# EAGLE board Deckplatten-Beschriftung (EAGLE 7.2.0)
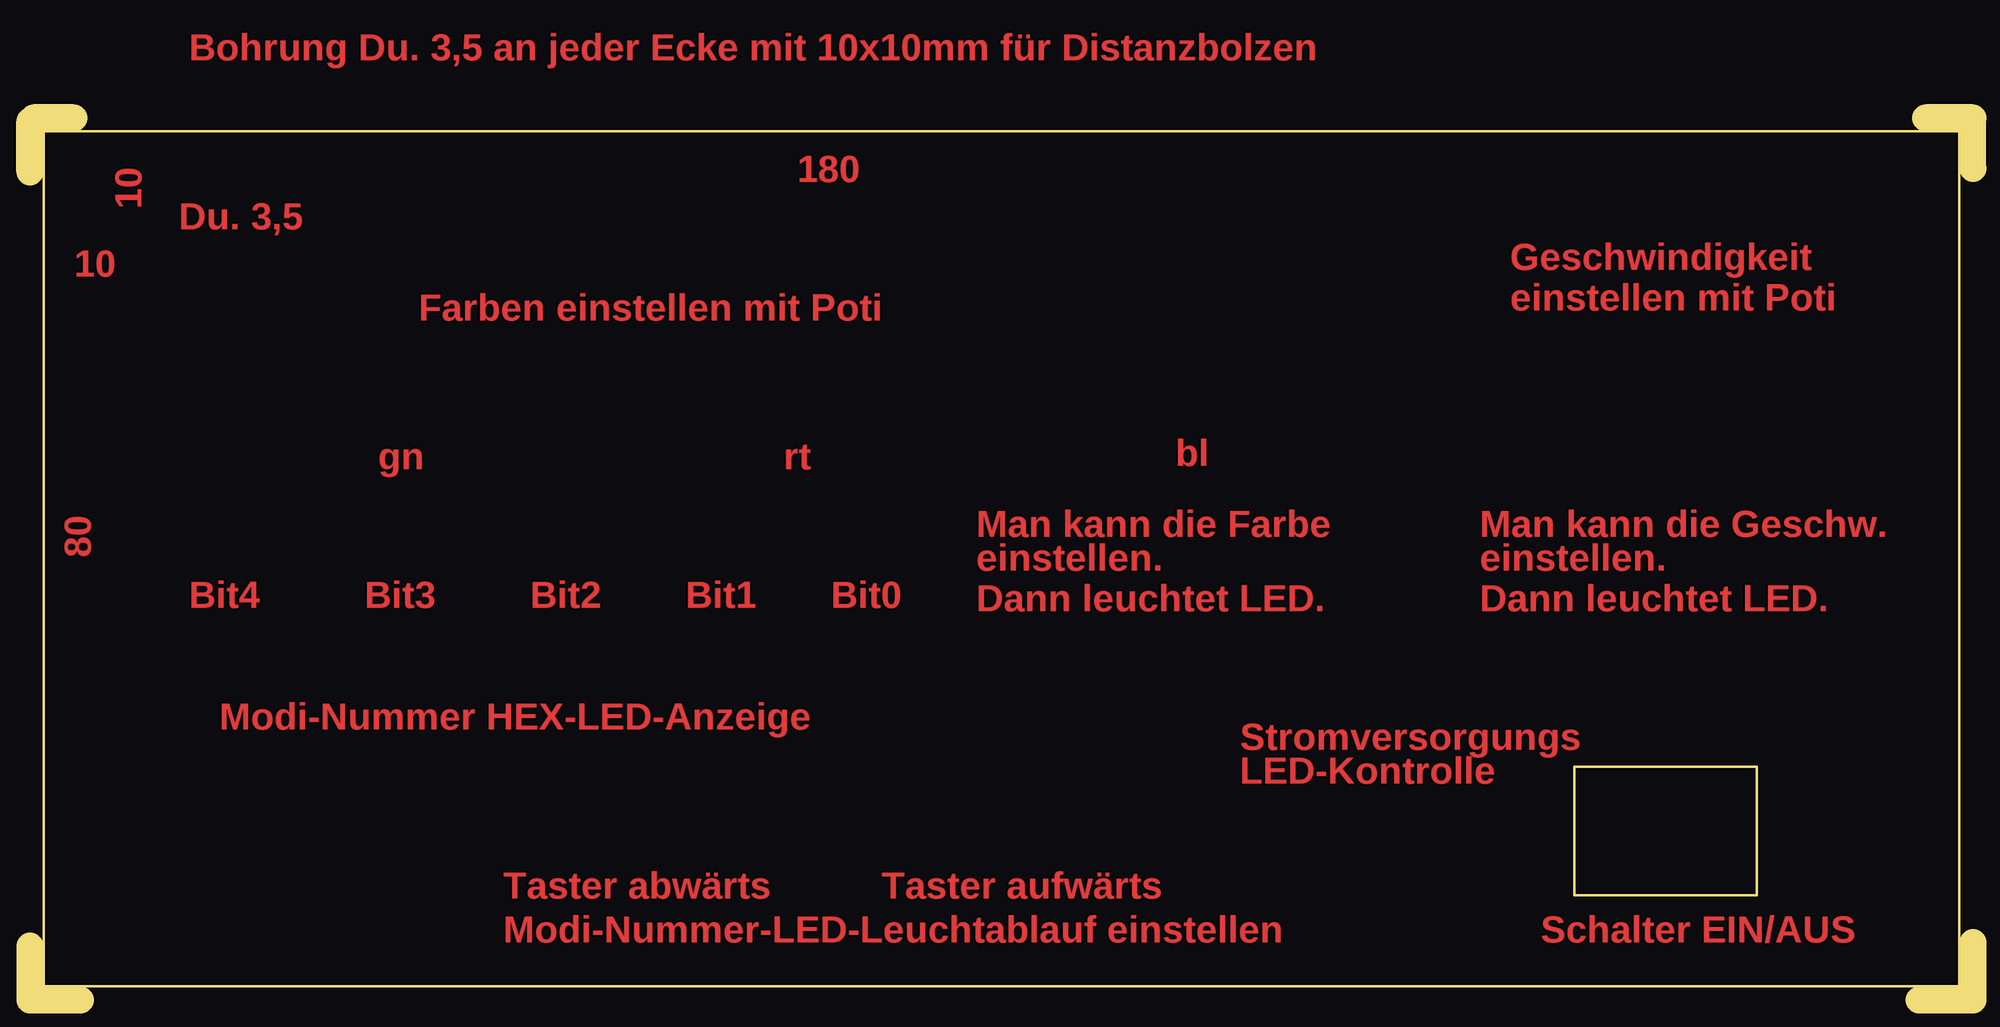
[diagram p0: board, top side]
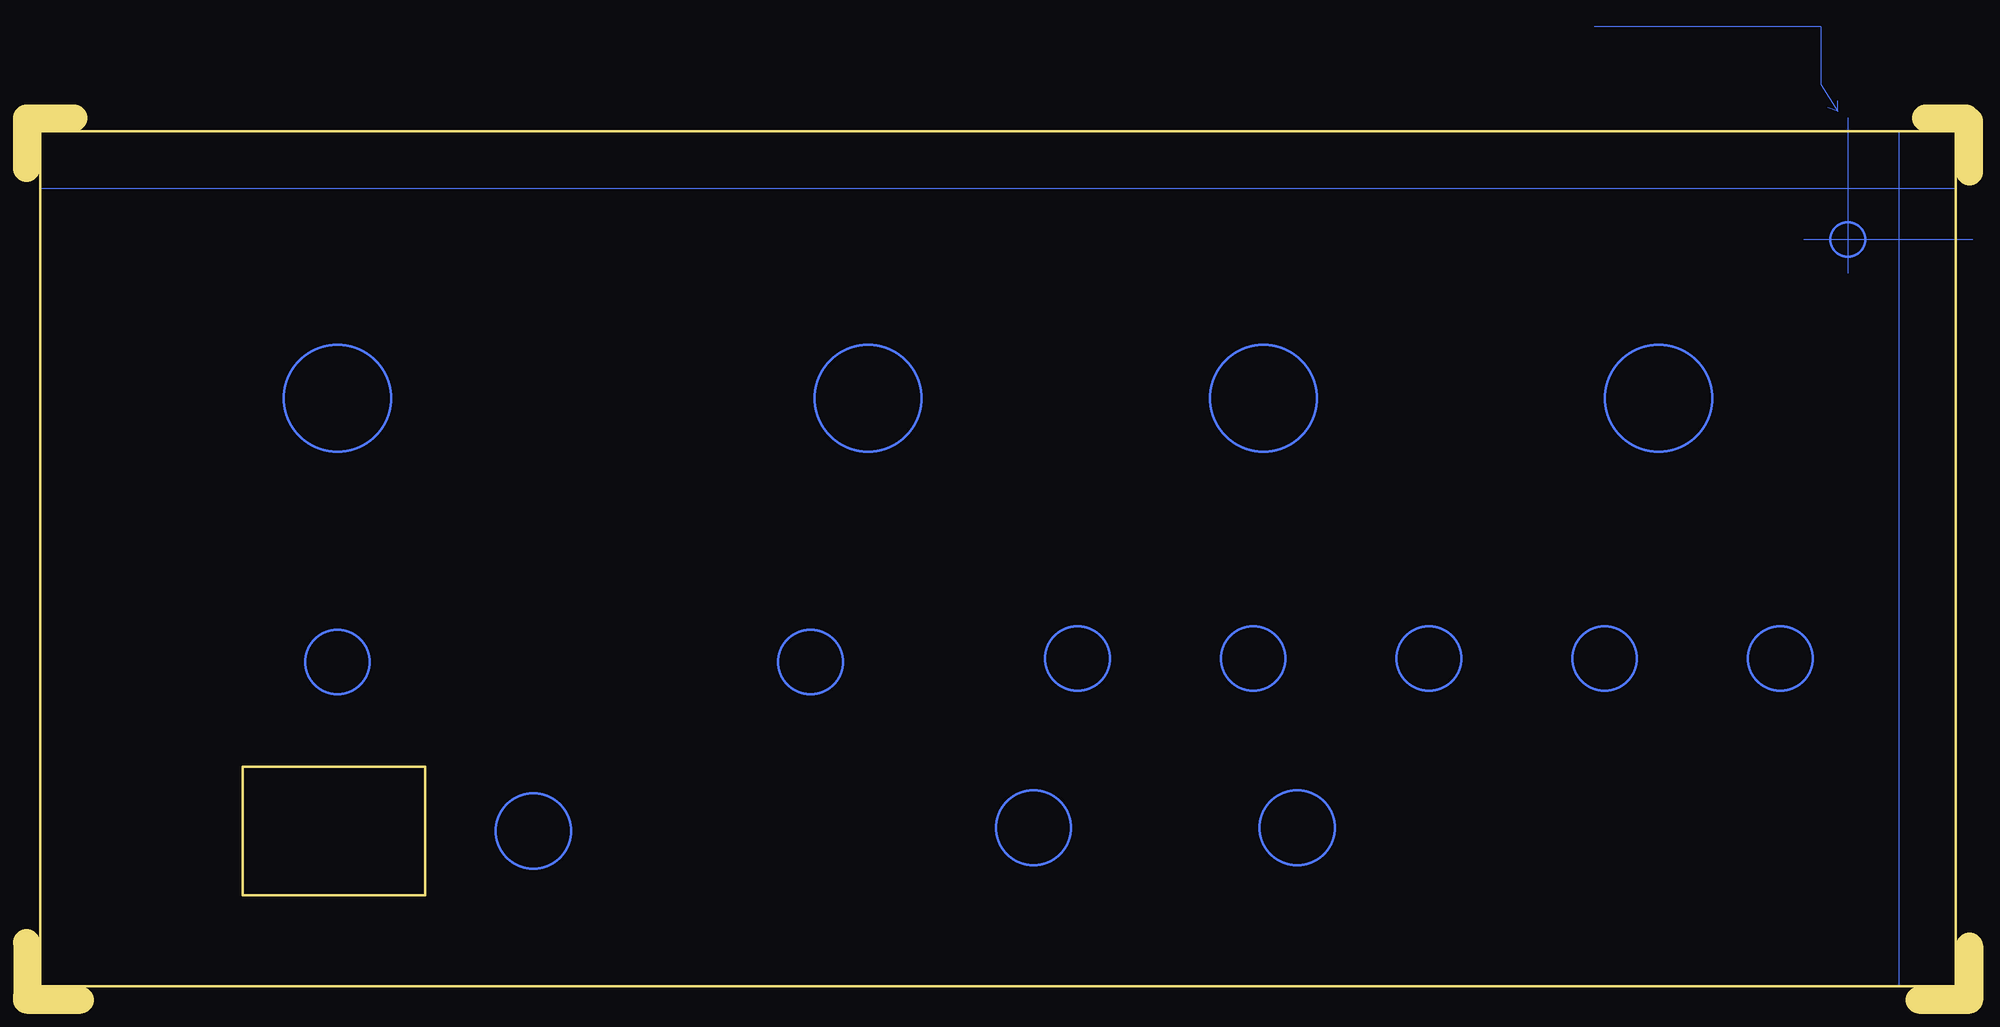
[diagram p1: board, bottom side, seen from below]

Size 182.56 x 82.87 mm. Coordinates in mm from the lower left corner, seen from the top.
Outline: 182.56,5.4 182.56,0.32
Outline: 182.56,0 177.48,0
Outline: 182.56,78.1 182.56,82.87 178.12,82.87
Outline: 0,5.08 0,0 4.76,0
Outline: 4.13,82.87 0.32,82.87
Outline: 0,77.79 0,82.55
Outline: 181.29,1.27 181.29,81.6 1.27,81.6 1.27,1.27 181.29,1.27
Outline: 162.24,21.91 162.24,9.84 145.1,9.84 145.1,21.91 162.24,21.91
Copper layers (1*16): Top 0.035mm / dielectric 1.5mm / Bottom 0.035mm
Design rules "default": minimum track width 10mil, minimum drill 24mil, track to track 8mil, track to pad 8mil, pad to pad 8mil, via to via 8mil, smd to smd 8mil, copper to edge 40mil, drill to drill 8mil, minimum pad ring 10mil, minimum via ring 8mil, stop-mask expansion 4mil, vias tented up to drill 0mil, thermal gap 10mil

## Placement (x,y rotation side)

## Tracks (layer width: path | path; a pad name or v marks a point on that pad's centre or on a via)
S$6
  Bottom 0: 1.27,64.77 1.27,64.14
S$7
  Bottom 0: 1.27,76.2 181.29,76.2
S$8
  Bottom 0: 6.67,81.6 6.67,1.27
S$18
  Bottom 0: 156.84,21.91 157.16,21.91
S$22
  Bottom 0: 11.43,82.87 11.43,68.26
S$23
  Bottom 0: -0.32,71.44 15.56,71.44
S$24
  Bottom 0: 12.38,83.5 13.97,86.04 13.97,91.44 35.24,91.44 | 12.38,83.5 13.33,83.82 | 12.38,83.5 12.38,84.45
(copper drawn outside any net)
  shapes: Bottom circle x15

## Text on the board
Top: Alles so ungefähr masstabs-getreu ! | Bohrung Du. 3,5 an jeder Ecke mit 10x10mm für Distanzbolzen | 180 | 10 | Du. 3,5 | 10 | Geschwindigkeit | einstellen mit Poti | Farben einstellen mit Poti | gn | rt | bl | Man kann die Farbe | Man kann die Geschw. | 80 | einstellen. | einstellen. | Bit4 | Bit3 | Bit2 | Bit1 | Bit0 | Dann leuchtet LED. | Dann leuchtet LED. | Modi-Nummer HEX-LED-Anzeige | Stromversorgungs | LED-Kontrolle | Taster abwärts | Taster aufwärts | Modi-Nummer-LED-Leuchtablauf einstellen | Schalter EIN/AUS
